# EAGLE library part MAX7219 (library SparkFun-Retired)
8-digit, 8-segment LED display driver, serial input
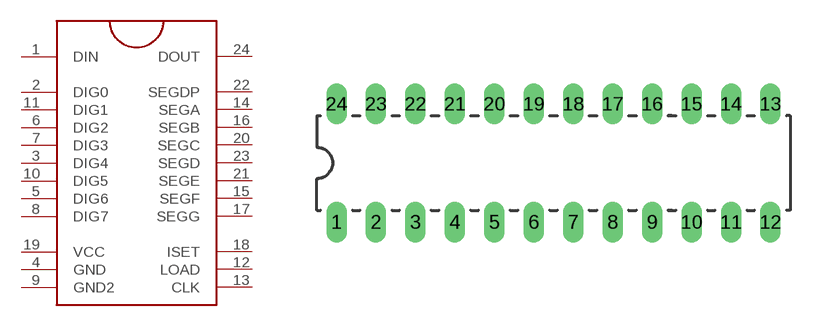
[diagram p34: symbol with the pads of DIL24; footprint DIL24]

Designator prefix -

## MAX7219DIP  [DIL24]
1  DIN
2  DIG0
3  DIG4
4  GND
5  DIG6
6  DIG2
7  DIG3
8  DIG7
9  GND2
10  DIG5
11  DIG1
12  LOAD
13  CLK
14  SEGA
15  SEGF
16  SEGB
17  SEGG
18  ISET
19  VCC
20  SEGC
21  SEGE
22  SEGDP
23  SEGD
24  DOUT

## Footprint DIL24 (pad centres in mm)
drill 0.813 long: 1 -13.97,-3.81; 2 -11.43,-3.81; 3 -8.89,-3.81; 4 -6.35,-3.81; 5 -3.81,-3.81; 6 -1.27,-3.81; 7 1.27,-3.81; 8 3.81,-3.81; 9 6.35,-3.81; 10 8.89,-3.81; 11 11.43,-3.81; 12 13.97,-3.81; 13 13.97,3.81; 14 11.43,3.81; 15 8.89,3.81; 16 6.35,3.81; 17 3.81,3.81; 18 1.27,3.81; 19 -1.27,3.81; 20 -3.81,3.81; 21 -6.35,3.81; 22 -8.89,3.81; 23 -11.43,3.81; 24 -13.97,3.81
